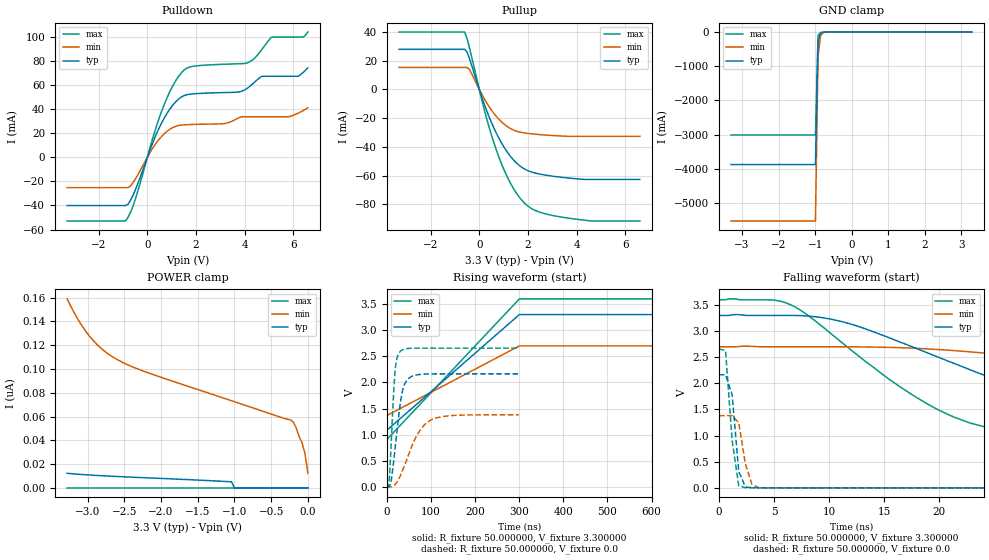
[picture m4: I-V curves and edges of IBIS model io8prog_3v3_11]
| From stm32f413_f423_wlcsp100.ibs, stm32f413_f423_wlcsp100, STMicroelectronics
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|   Model io8prog_3v3_11
[Model]  io8prog_3v3_11
Model_type I/O
Polarity   Non-Inverting
Enable   Active-Low
Vinl =   0.990000V
Vinh =   2.310000V
Vmeas =  1.650000V
Cref =   100.000000nF
Rref =   1.000000k
Vref =   3.300000V
C_comp   2.665600pF   2.506300pF   2.859000pF
[Temperature Range]   25.000000   0.125000k   -40.000000
[Pullup Reference]   3.300000V   2.700000V   3.600000V
[Pulldown Reference]   0.0V   0.0V   0.0V
[POWER Clamp Reference]   3.300000V   2.700000V   3.600000V
[GND Clamp Reference]   0.0V   0.0V   0.0V
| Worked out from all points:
|   slope of the pulldown table from 0 to 0.495 V, typ, clamps not added: 20 ohm
|   slope of the pullup table from 0 to 0.495 V, typ, clamps not added: 21.7 ohm
|   GND clamp passes 1 mA (typ) near -0.57 V on its own axis
|   rising waveform, R_fixture 50.000000, V_fixture 3.300000: 20-80 % time 180ns typ, 180ns min, 180ns max; typ from 1.09 V to 3.3 V
|   rising waveform, R_fixture 50.000000, V_fixture 0.0: 20-80 % time 18.3ns typ, 43.3ns min, 9.74ns max; typ from 0 V to 2.17 V
|   falling waveform, R_fixture 50.000000, V_fixture 3.300000: 20-80 % time 17.4ns typ, 34.6ns min, 10.8ns max; typ from 3.3 V to 1.09 V
|   falling waveform, R_fixture 50.000000, V_fixture 0.0: 20-80 % time 530ps typ, 770ps min, 682ps max; typ from 2.17 V to 0 V
[Pulldown]
|Voltage   I(typ)   I(min)   I(max)
-3.3V     -40.11mA   -25.24mA   -52.93mA
-900mV    -40.11mA   -25.24mA   -52.93mA
-500mV    -27.39mA   -18.31mA   -35.21mA
600mV     29.01mA    17.61mA    38.88mA
1.1V      44.56mA    25.16mA    61.26mA
1.5V      51.11mA    26.89mA    72.21mA
3.1V      53.67mA    27.79mA    77.15mA
4.1V      57.11mA    33.57mA    78.25mA
4.7V      67.22mA    33.57mA    89.26mA
5.1V      67.22mA    33.57mA    99.69mA
6.2V      67.22mA    36.63mA    99.69mA
6.6V      74.18mA    41.08mA    104mA
[Pullup]
|Voltage   I(typ)   I(min)   I(max)
-3.3V     27.94mA    15.3mA     39.98mA
-600mV    27.94mA    15.3mA     39.98mA
-500mV    25.89mA    15.3mA     35.29mA
-400mV    21.3mA     13.82mA    28.75mA
300mV     -14.62mA   -9.248mA   -20.15mA
800mV     -33.8mA    -20.67mA   -46.89mA
1.1V      -42.41mA   -25.28mA   -59.19mA
1.4V      -49.01mA   -28.29mA   -68.91mA
2V        -56.64mA   -30.64mA   -81.32mA
2.6V      -59.37mA   -31.63mA   -86.14mA
3.9V      -62.11mA   -32.7mA    -90.25mA
6.6V      -62.7mA    -32.7mA    -91.7mA
[GND_clamp]
|Voltage   I(typ)   I(min)   I(max)
-3.3V     -3.872A    -5.523A    -3.009A
-990mV    -3.872A    -5.523A    -3.009A
-920mV    -262.2mA   -719.6mA   -104.3mA
-850mV    -25.19mA   -100.9mA   -13.07mA
-780mV    -6.959mA   -18mA      -7.19mA
3.28V     0A         5.62nA     0A
[POWER_clamp]
|Voltage   I(typ)   I(min)   I(max)
-3.28V    12.27nA    159nA      0A
-3.12V    11.41nA    140.5nA    0A
-2.96V    10.73nA    126.5nA    0A
-2.76V    10.05nA    114.5nA    0A
-2.56V    9.455nA    106.7nA    0A
-1.04V    5.085nA    73.31nA    0A
-1V       0A         72.48nA    0A
-240mV    0A         57.24nA    0A
-200mV    0A         55.42nA    0A
-80mV     0A         37.96nA    0A
-40mV     0A         28.96nA    0A
0V        0A         12.44nA    0A
[Ramp]
| variable   typ   min   max
dV/dt_r  1.29876/18.26930n   0.82878/43.28389n   1.59366/9.73351n
dV/dt_f  1.32768/17.42868n   0.79902/35.60785n   1.61434/10.81937n
R_load = 50.000000
[Rising Waveform]
R_fixture= 50.000000
V_fixture= 3.300000
V_fixture_min= 2.700000
V_fixture_max= 3.600000
|time   V(typ)   V(min)   V(max)
0s        1.087V     1.368V     909.4mV
300.3ns   3.3V       2.7V       3.6V
600.6ns   3.3V       2.7V       3.6V
29.73us   3.3V       2.7V       3.6V
[Rising Waveform]
R_fixture= 50.000000
V_fixture= 0.0
V_fixture_min= 0.0
V_fixture_max= 0.0
|time   V(typ)   V(min)   V(max)
0s        -514.1nV   -456.8nV   816.9nV
5.405ns   9.883mV    -123.4uV   167.6mV
10.21ns   156.6mV    2.373mV    959.1mV
18.62ns   756.7mV    50.31mV    2.243V
30.63ns   1.625V     221.3mV    2.599V
37.84ns   1.921V     368.4mV    2.634V
49.85ns   2.083V     636.6mV    2.651V
70.87ns   2.149V     1.031V     2.656V
98.5ns    2.162V     1.276V     2.656V
299.1ns   2.165V     1.381V     2.656V
[Falling Waveform]
R_fixture= 50.000000
V_fixture= 3.300000
V_fixture_min= 2.700000
V_fixture_max= 3.600000
|time   V(typ)   V(min)   V(max)
0s        3.3V       2.7V       3.6V
6.607ns   3.3V       2.7V       3.495V
11.41ns   3.169V     2.7V       2.737V
19.82ns   2.508V     2.649V     1.501V
24.02ns   2.159V     2.581V     1.173V
27.93ns   1.853V     2.494V     1.062V
33.63ns   1.502V     2.35V      995.1mV
40.54ns   1.299V     2.162V     956.9mV
70.27ns   1.123V     1.579V     915.2mV
149.5ns   1.087V     1.368V     909.4mV
[Falling Waveform]
R_fixture= 50.000000
V_fixture= 0.0
V_fixture_min= 0.0
V_fixture_max= 0.0
|time   V(typ)   V(min)   V(max)
0s        2.165V     1.381V     2.656V
600.6ps   2.165V     1.381V     2.632V
1.201ns   1.782V     1.382V     903.8mV
1.802ns   309.6mV    1.246V     36.45mV
2.402ns   17.85mV    460.6mV    3.121mV
3.003ns   2.49mV     61.26mV    1.584mV
3.604ns   1.219mV    6.567mV    1.176mV
4.204ns   924.5uV    1.605mV    940uV
299.1ns   -514.1nV   -456.8nV   816.9nV
